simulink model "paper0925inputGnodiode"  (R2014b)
settings: Solver=ode15s  StartTime=0.0  StopTime=24  FixedStep=1e-4  RelTol=1e-3
libraries: nesl_utility x19, elec_lib x16, fl_lib x3

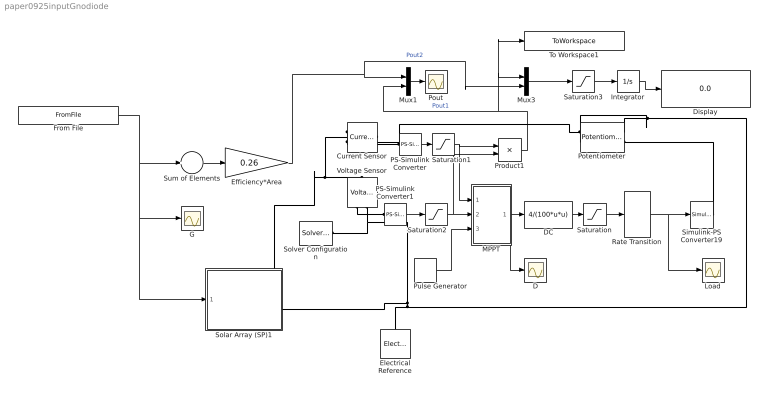
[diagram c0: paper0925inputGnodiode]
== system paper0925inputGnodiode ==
  Current Sensor : fl_lib/Electrical/Electrical Sensors/Current Sensor
  D : Scope
  DC : Fcn  Expr=4/(100*u*u)
  Display : Display
  Efficiency*Area : Gain  Gain=0.26
  Electrical Reference : fl_lib/Electrical/Electrical Elements/Electrical Reference
  From File : FromFile  FileName=Goverlap0_3.mat  SampleTime=0
  G : Scope
  Integrator : Integrator
  Load : Scope
  MPPT : Subsystem
  Mux1 : Mux  Inputs=2
  Mux3 : Mux  Inputs=2
  PS-Simulink Converter : nesl_utility/PS-Simulink Converter  PhysicalDomain=network_engine_domain  SubClassName=ps_output  LeftPortType=input  RightPortType=output  PseudoPeriodic=off  Frequencies=[]  Unit=1  AffineConversion=off
  PS-Simulink Converter1 : nesl_utility/PS-Simulink Converter  PhysicalDomain=network_engine_domain  SubClassName=ps_output  LeftPortType=input  RightPortType=output  PseudoPeriodic=off  Frequencies=[]  Unit=1  AffineConversion=off
  Potentiometer : elec_lib/Passive Devices/Potentiometer  R0=100 Ohm  Rw=0.01 Ohm  Rcenter=200 Ohm  xmin=0  xmax=1  Taper=1  Gradient=1  xminL=0  xmaxL=1  lambda=1  A=1 Ohm
  Pout : Scope
  Product1 : Product
  Pulse Generator : DiscretePulseGenerator  PulseType=Time based  Period=0.5  PulseWidth=0.1
  Rate Transition : RateTransition
  Saturation : Saturate  UpperLimit=1  LowerLimit=0
  Saturation1 : Saturate  UpperLimit=40  LowerLimit=0
  Saturation2 : Saturate  UpperLimit=500  LowerLimit=0
  Saturation3 : Saturate  UpperLimit=6000  LowerLimit=0
  Simulink-PS Converter19 : nesl_utility/Simulink-PS Converter  PhysicalDomain=network_engine_domain  SubClassName=ps_input  LeftPortType=input  RightPortType=output  PseudoPeriodic=off  Frequencies=[]  NoiseDistribution=none  NoiseParameters=[]  Unit=1  AffineConversion=off  InputFiltering=off  SimscapeFilterOrder=1  InputFilterTimeConstant=0.001  UdotUserProvided=1
  Solar Array (SP)1 : Subsystem
  Solver Configuration : nesl_utility/Solver Configuration  PhysicalDomain=network_engine_domain  SubClassName=solver  LeftPortType=input  RightPortType=generic  Accelerate=off  Tones=[]  Harmonics=[]  SimulateNoise=off  Profile=off  UseLocalSampling=off  EnableSwitchedLinearOptims=on  FrequencyDomain=off  UseCCode=off  RelTol=0.001  AbsTol=1e-06  MinStep=1e-09  ToWorkspace=off  DoDC=off  ResidualTolerance=1e-9  UseLocalSolver=on  LocalSolverChoice=NE_BACKWARD_EULER_ADVANCER  LocalSolverSampleTime=1e-4  DoFixedCost=on  MaxNonlinIter=3  MaxModeIter=2  LinearAlgebra=Sparse  DelaysMemoryBudget=1024  AutomaticFiltering=on  FilteringTimeConstant=0.001
  Sum of Elements : Sum  Inputs=+
  To Workspace1 : ToWorkspace  VariableName=Poverlap0_3SPnodiode  SampleTime=-1
  Voltage Sensor : fl_lib/Electrical/Electrical Sensors/Voltage Sensor
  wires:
  Sum of Elements/1 -> Efficiency*Area/1
  PS-Simulink Converter/1 -> Saturation1/1
  Product1/1 -> Mux3/1, To Workspace1/1, Mux1/2  "Pout1"
  PS-Simulink Converter1/1 -> Saturation2/1
  DC/1 -> Saturation/1
  Saturation/1 -> Rate Transition/1
  MPPT/1(D) -> D/1, DC/1
  Pulse Generator/1 -> MPPT/3(Control)
  Mux1/1 -> Pout/1
  Efficiency*Area/1 -> Mux3/2, Mux1/1  "Pout2"
  Mux3/1 -> Saturation3/1
  Rate Transition/1 -> Load/1, Simulink-PS Converter19/1
  From File/1 -> Solar Array (SP)1/1(G), G/1, Sum of Elements/1
  Saturation1/1 -> Product1/1, MPPT/1(I)
  Saturation2/1 -> Product1/2, MPPT/2(V)
  Saturation3/1 -> Integrator/1
  Integrator/1 -> Display/1
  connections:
  Voltage Sensor/LConn1 -- Solar Array (SP)1/RConn1 -- Current Sensor/LConn1
  Voltage Sensor/RConn2 -- Solar Array (SP)1/RConn2 -- Electrical Reference/LConn1 -- Potentiometer/LConn2 -- Potentiometer/RConn1 -- Solver Configuration/RConn1
  Current Sensor/RConn1 -- PS-Simulink Converter/LConn1
  Voltage Sensor/RConn1 -- PS-Simulink Converter1/LConn1
  Simulink-PS Converter19/RConn1 -- Potentiometer/RConn2
  Potentiometer/LConn1 -- Current Sensor/RConn2

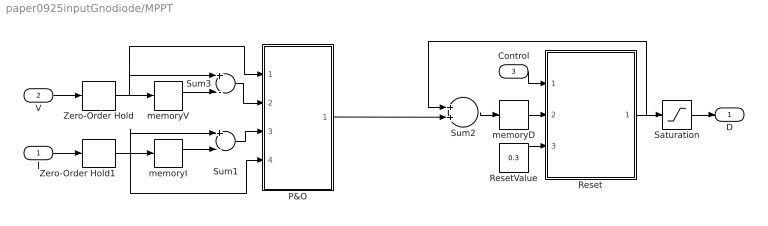
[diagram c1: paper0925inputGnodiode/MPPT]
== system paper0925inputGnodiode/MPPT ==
  I : Inport
  V : Inport  Port=2
  Control : Inport  Port=3
  P&O : MATLAB Function  TreatAsAtomicUnit=on
  Reset : MATLAB Function  TreatAsAtomicUnit=on
  ResetValue : Constant  Value=0.3
  Saturation : Saturate  UpperLimit=1  LowerLimit=1e-9
  Sum1 : Sum  Inputs=+-
  Sum2 : Sum  Inputs=2
  Sum3 : Sum  Inputs=+-
  Zero-Order Hold : ZeroOrderHold  SampleTime=1e-3
  Zero-Order Hold1 : ZeroOrderHold  SampleTime=1e-3
  memoryD : Memory  X0=0.3  InheritSampleTime=on
  memoryI : Memory  InheritSampleTime=on
  memoryV : Memory  InheritSampleTime=on
  D : Outport
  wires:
  Sum2/1 -> memoryD/1
  V/1 -> Zero-Order Hold/1
  I/1 -> Zero-Order Hold1/1
  Zero-Order Hold/1 -> P&O/1(V), Sum3/1, memoryV/1
  memoryV/1 -> Sum3/2
  Zero-Order Hold1/1 -> Sum1/1, P&O/4(I), memoryI/1
  memoryI/1 -> Sum1/2
  Saturation/1 -> D/1
  Sum3/1 -> P&O/2(dV)
  Sum1/1 -> P&O/3(dI)
  P&O/1(dD) -> Sum2/2
  ResetValue/1 -> Reset/3(ResetValue)
  memoryD/1 -> Reset/2(in)
  Reset/1(out) -> Sum2/1, Saturation/1
  Control/1 -> Reset/1(control)

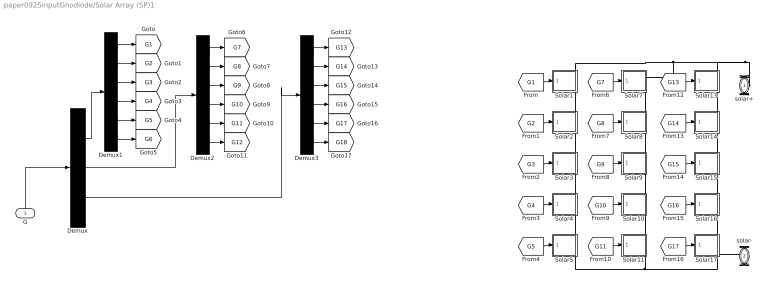
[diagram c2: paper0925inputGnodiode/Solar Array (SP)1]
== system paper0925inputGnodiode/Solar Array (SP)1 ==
  G : Inport
  Demux : Demux  Outputs=3
  Demux1 : Demux  Outputs=6
  Demux2 : Demux  Outputs=6
  Demux3 : Demux  Outputs=6
  Solar1 : Subsystem
  Solar10 : Subsystem
  Solar11 : Subsystem
  Solar13 : Subsystem
  Solar14 : Subsystem
  Solar15 : Subsystem
  Solar16 : Subsystem
  Solar17 : Subsystem
  Solar2 : Subsystem
  Solar3 : Subsystem
  Solar4 : Subsystem
  Solar5 : Subsystem
  Solar7 : Subsystem
  Solar8 : Subsystem
  Solar9 : Subsystem
  solar+ : PMIOPort  Port=1  Side=Right
  solar- : PMIOPort  Port=2  Side=Right
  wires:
  [G1] -> Solar1/1(G)
  [G2] -> Solar2/1(G)
  [G3] -> Solar3/1(G)
  G/1 -> Demux/1
  [G4] -> Solar4/1(G)
  [G5] -> Solar5/1(G)
  [G7] -> Solar7/1(G)
  [G8] -> Solar8/1(G)
  [G9] -> Solar9/1(G)
  [G10] -> Solar10/1(G)
  [G11] -> Solar11/1(G)
  [G13] -> Solar13/1(G)
  [G14] -> Solar14/1(G)
  [G15] -> Solar15/1(G)
  [G16] -> Solar16/1(G)
  [G17] -> Solar17/1(G)
  Demux/1 -> Demux1/1
  Demux1/1 -> [G1]
  Demux1/2 -> [G2]
  Demux1/3 -> [G3]
  Demux1/4 -> [G4]
  Demux1/5 -> [G5]
  Demux1/6 -> [G6]
  Demux/2 -> Demux2/1
  Demux/3 -> Demux3/1
  Demux2/1 -> [G7]
  Demux2/2 -> [G8]
  Demux2/3 -> [G9]
  Demux2/4 -> [G10]
  Demux2/5 -> [G11]
  Demux2/6 -> [G12]
  Demux3/1 -> [G13]
  Demux3/2 -> [G14]
  Demux3/3 -> [G15]
  Demux3/4 -> [G16]
  Demux3/5 -> [G17]
  Demux3/6 -> [G18]
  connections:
  Solar15/RConn2 -- Solar16/RConn1
  Solar13/RConn2 -- Solar14/RConn1
  Solar8/RConn2 -- Solar9/RConn1
  Solar4/RConn2 -- Solar5/RConn1
  Solar5/RConn2 -- Solar11/RConn2 -- Solar17/RConn2 -- solar-/RConn1
  solar+/RConn1 -- Solar1/RConn1 -- Solar7/RConn1 -- Solar13/RConn1
  Solar1/RConn2 -- Solar2/RConn1
  Solar7/RConn2 -- Solar8/RConn1
  Solar14/RConn2 -- Solar15/RConn1
  Solar2/RConn2 -- Solar3/RConn1
  Solar3/RConn2 -- Solar4/RConn1
  Solar9/RConn2 -- Solar10/RConn1
  Solar16/RConn2 -- Solar17/RConn1
  Solar10/RConn2 -- Solar11/RConn1

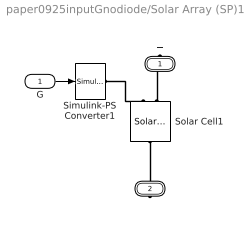
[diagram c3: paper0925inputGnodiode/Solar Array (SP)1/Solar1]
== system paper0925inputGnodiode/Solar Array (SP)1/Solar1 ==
  G : Inport
  Simulink-PS Converter1 : nesl_utility/Simulink-PS Converter  PhysicalDomain=network_engine_domain  SubClassName=ps_input  LeftPortType=input  RightPortType=output  PseudoPeriodic=off  Frequencies=[]  NoiseDistribution=none  NoiseParameters=[]  Unit=1  AffineConversion=off  InputFiltering=off  SimscapeFilterOrder=1  InputFilterTimeConstant=0.001  UdotUserProvided=1
  Solar Cell1 : elec_lib/Sources/Solar Cell  prm=1  Isc=7.34 A  Voc=0.6 V  Is=1e-6 A  Is2=0 A  Iph=7.34 A  Ir0=1000 W/m^2  ec=1.2  N2=2  Rs=1e-3 Ohm  Rp=Inf Ohm  N_series=90  TIPH1=0 1/K  EG=1.11 eV  TXIS1=3  TXIS2=3  TRS1=0  TRP1=0  Tmeas=25 C  TFIXED=25 C  thermal_mass=100 J/K  initial_temperature=25 C
  + : PMIOPort  Port=1  Side=Right
  - : PMIOPort  Port=2  Side=Right
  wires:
  G/1 -> Simulink-PS Converter1/1
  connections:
  Simulink-PS Converter1/RConn1 -- Solar Cell1/LConn1
  Solar Cell1/LConn2 -- +/RConn1
  Solar Cell1/RConn1 -- -/RConn1

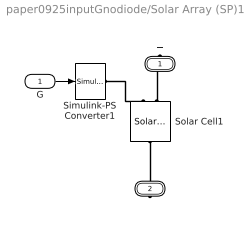
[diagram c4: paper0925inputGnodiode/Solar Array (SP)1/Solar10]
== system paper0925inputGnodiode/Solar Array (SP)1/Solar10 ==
  G : Inport
  Simulink-PS Converter1 : nesl_utility/Simulink-PS Converter  PhysicalDomain=network_engine_domain  SubClassName=ps_input  LeftPortType=input  RightPortType=output  PseudoPeriodic=off  Frequencies=[]  NoiseDistribution=none  NoiseParameters=[]  Unit=1  AffineConversion=off  InputFiltering=off  SimscapeFilterOrder=1  InputFilterTimeConstant=0.001  UdotUserProvided=1
  Solar Cell1 : elec_lib/Sources/Solar Cell  prm=1  Isc=7.34 A  Voc=0.6 V  Is=1e-6 A  Is2=0 A  Iph=7.34 A  Ir0=1000 W/m^2  ec=1.2  N2=2  Rs=1e-3 Ohm  Rp=Inf Ohm  N_series=90  TIPH1=0 1/K  EG=1.11 eV  TXIS1=3  TXIS2=3  TRS1=0  TRP1=0  Tmeas=25 C  TFIXED=25 C  thermal_mass=100 J/K  initial_temperature=25 C
  + : PMIOPort  Port=1  Side=Right
  - : PMIOPort  Port=2  Side=Right
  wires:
  G/1 -> Simulink-PS Converter1/1
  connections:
  Simulink-PS Converter1/RConn1 -- Solar Cell1/LConn1
  Solar Cell1/LConn2 -- +/RConn1
  Solar Cell1/RConn1 -- -/RConn1

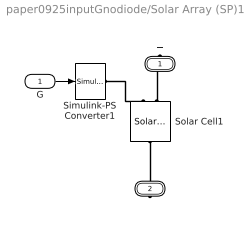
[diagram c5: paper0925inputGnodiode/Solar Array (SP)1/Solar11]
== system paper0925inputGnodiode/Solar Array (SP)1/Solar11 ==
  G : Inport
  Simulink-PS Converter1 : nesl_utility/Simulink-PS Converter  PhysicalDomain=network_engine_domain  SubClassName=ps_input  LeftPortType=input  RightPortType=output  PseudoPeriodic=off  Frequencies=[]  NoiseDistribution=none  NoiseParameters=[]  Unit=1  AffineConversion=off  InputFiltering=off  SimscapeFilterOrder=1  InputFilterTimeConstant=0.001  UdotUserProvided=1
  Solar Cell1 : elec_lib/Sources/Solar Cell  prm=1  Isc=7.34 A  Voc=0.6 V  Is=1e-6 A  Is2=0 A  Iph=7.34 A  Ir0=1000 W/m^2  ec=1.2  N2=2  Rs=1e-3 Ohm  Rp=Inf Ohm  N_series=90  TIPH1=0 1/K  EG=1.11 eV  TXIS1=3  TXIS2=3  TRS1=0  TRP1=0  Tmeas=25 C  TFIXED=25 C  thermal_mass=100 J/K  initial_temperature=25 C
  + : PMIOPort  Port=1  Side=Right
  - : PMIOPort  Port=2  Side=Right
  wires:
  G/1 -> Simulink-PS Converter1/1
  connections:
  Simulink-PS Converter1/RConn1 -- Solar Cell1/LConn1
  Solar Cell1/LConn2 -- +/RConn1
  Solar Cell1/RConn1 -- -/RConn1

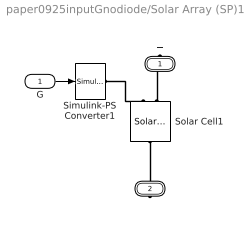
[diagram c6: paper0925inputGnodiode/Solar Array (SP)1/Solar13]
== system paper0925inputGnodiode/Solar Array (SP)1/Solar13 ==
  G : Inport
  Simulink-PS Converter1 : nesl_utility/Simulink-PS Converter  PhysicalDomain=network_engine_domain  SubClassName=ps_input  LeftPortType=input  RightPortType=output  PseudoPeriodic=off  Frequencies=[]  NoiseDistribution=none  NoiseParameters=[]  Unit=1  AffineConversion=off  InputFiltering=off  SimscapeFilterOrder=1  InputFilterTimeConstant=0.001  UdotUserProvided=1
  Solar Cell1 : elec_lib/Sources/Solar Cell  prm=1  Isc=7.34 A  Voc=0.6 V  Is=1e-6 A  Is2=0 A  Iph=7.34 A  Ir0=1000 W/m^2  ec=1.2  N2=2  Rs=1e-3 Ohm  Rp=Inf Ohm  N_series=90  TIPH1=0 1/K  EG=1.11 eV  TXIS1=3  TXIS2=3  TRS1=0  TRP1=0  Tmeas=25 C  TFIXED=25 C  thermal_mass=100 J/K  initial_temperature=25 C
  + : PMIOPort  Port=1  Side=Right
  - : PMIOPort  Port=2  Side=Right
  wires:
  G/1 -> Simulink-PS Converter1/1
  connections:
  Simulink-PS Converter1/RConn1 -- Solar Cell1/LConn1
  Solar Cell1/LConn2 -- +/RConn1
  Solar Cell1/RConn1 -- -/RConn1

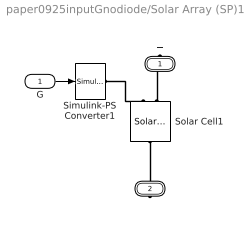
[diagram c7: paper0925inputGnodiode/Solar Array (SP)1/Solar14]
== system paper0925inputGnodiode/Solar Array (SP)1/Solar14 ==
  G : Inport
  Simulink-PS Converter1 : nesl_utility/Simulink-PS Converter  PhysicalDomain=network_engine_domain  SubClassName=ps_input  LeftPortType=input  RightPortType=output  PseudoPeriodic=off  Frequencies=[]  NoiseDistribution=none  NoiseParameters=[]  Unit=1  AffineConversion=off  InputFiltering=off  SimscapeFilterOrder=1  InputFilterTimeConstant=0.001  UdotUserProvided=1
  Solar Cell1 : elec_lib/Sources/Solar Cell  prm=1  Isc=7.34 A  Voc=0.6 V  Is=1e-6 A  Is2=0 A  Iph=7.34 A  Ir0=1000 W/m^2  ec=1.2  N2=2  Rs=1e-3 Ohm  Rp=Inf Ohm  N_series=90  TIPH1=0 1/K  EG=1.11 eV  TXIS1=3  TXIS2=3  TRS1=0  TRP1=0  Tmeas=25 C  TFIXED=25 C  thermal_mass=100 J/K  initial_temperature=25 C
  + : PMIOPort  Port=1  Side=Right
  - : PMIOPort  Port=2  Side=Right
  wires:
  G/1 -> Simulink-PS Converter1/1
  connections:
  Simulink-PS Converter1/RConn1 -- Solar Cell1/LConn1
  Solar Cell1/LConn2 -- +/RConn1
  Solar Cell1/RConn1 -- -/RConn1

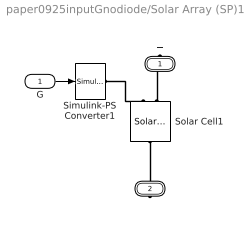
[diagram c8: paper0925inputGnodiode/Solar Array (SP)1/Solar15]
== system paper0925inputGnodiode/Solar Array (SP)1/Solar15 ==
  G : Inport
  Simulink-PS Converter1 : nesl_utility/Simulink-PS Converter  PhysicalDomain=network_engine_domain  SubClassName=ps_input  LeftPortType=input  RightPortType=output  PseudoPeriodic=off  Frequencies=[]  NoiseDistribution=none  NoiseParameters=[]  Unit=1  AffineConversion=off  InputFiltering=off  SimscapeFilterOrder=1  InputFilterTimeConstant=0.001  UdotUserProvided=1
  Solar Cell1 : elec_lib/Sources/Solar Cell  prm=1  Isc=7.34 A  Voc=0.6 V  Is=1e-6 A  Is2=0 A  Iph=7.34 A  Ir0=1000 W/m^2  ec=1.2  N2=2  Rs=1e-3 Ohm  Rp=Inf Ohm  N_series=90  TIPH1=0 1/K  EG=1.11 eV  TXIS1=3  TXIS2=3  TRS1=0  TRP1=0  Tmeas=25 C  TFIXED=25 C  thermal_mass=100 J/K  initial_temperature=25 C
  + : PMIOPort  Port=1  Side=Right
  - : PMIOPort  Port=2  Side=Right
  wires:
  G/1 -> Simulink-PS Converter1/1
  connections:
  Simulink-PS Converter1/RConn1 -- Solar Cell1/LConn1
  Solar Cell1/LConn2 -- +/RConn1
  Solar Cell1/RConn1 -- -/RConn1

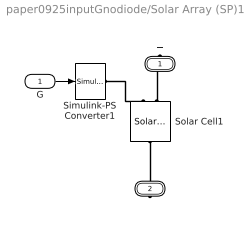
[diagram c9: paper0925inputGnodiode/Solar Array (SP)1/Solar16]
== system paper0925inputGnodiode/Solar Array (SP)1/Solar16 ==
  G : Inport
  Simulink-PS Converter1 : nesl_utility/Simulink-PS Converter  PhysicalDomain=network_engine_domain  SubClassName=ps_input  LeftPortType=input  RightPortType=output  PseudoPeriodic=off  Frequencies=[]  NoiseDistribution=none  NoiseParameters=[]  Unit=1  AffineConversion=off  InputFiltering=off  SimscapeFilterOrder=1  InputFilterTimeConstant=0.001  UdotUserProvided=1
  Solar Cell1 : elec_lib/Sources/Solar Cell  prm=1  Isc=7.34 A  Voc=0.6 V  Is=1e-6 A  Is2=0 A  Iph=7.34 A  Ir0=1000 W/m^2  ec=1.2  N2=2  Rs=1e-3 Ohm  Rp=Inf Ohm  N_series=90  TIPH1=0 1/K  EG=1.11 eV  TXIS1=3  TXIS2=3  TRS1=0  TRP1=0  Tmeas=25 C  TFIXED=25 C  thermal_mass=100 J/K  initial_temperature=25 C
  + : PMIOPort  Port=1  Side=Right
  - : PMIOPort  Port=2  Side=Right
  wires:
  G/1 -> Simulink-PS Converter1/1
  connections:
  Simulink-PS Converter1/RConn1 -- Solar Cell1/LConn1
  Solar Cell1/LConn2 -- +/RConn1
  Solar Cell1/RConn1 -- -/RConn1

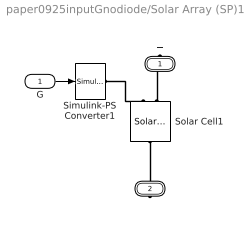
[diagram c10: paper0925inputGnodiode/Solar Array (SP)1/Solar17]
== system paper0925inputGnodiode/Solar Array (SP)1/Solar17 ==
  G : Inport
  Simulink-PS Converter1 : nesl_utility/Simulink-PS Converter  PhysicalDomain=network_engine_domain  SubClassName=ps_input  LeftPortType=input  RightPortType=output  PseudoPeriodic=off  Frequencies=[]  NoiseDistribution=none  NoiseParameters=[]  Unit=1  AffineConversion=off  InputFiltering=off  SimscapeFilterOrder=1  InputFilterTimeConstant=0.001  UdotUserProvided=1
  Solar Cell1 : elec_lib/Sources/Solar Cell  prm=1  Isc=7.34 A  Voc=0.6 V  Is=1e-6 A  Is2=0 A  Iph=7.34 A  Ir0=1000 W/m^2  ec=1.2  N2=2  Rs=1e-3 Ohm  Rp=Inf Ohm  N_series=90  TIPH1=0 1/K  EG=1.11 eV  TXIS1=3  TXIS2=3  TRS1=0  TRP1=0  Tmeas=25 C  TFIXED=25 C  thermal_mass=100 J/K  initial_temperature=25 C
  + : PMIOPort  Port=1  Side=Right
  - : PMIOPort  Port=2  Side=Right
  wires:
  G/1 -> Simulink-PS Converter1/1
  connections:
  Simulink-PS Converter1/RConn1 -- Solar Cell1/LConn1
  Solar Cell1/LConn2 -- +/RConn1
  Solar Cell1/RConn1 -- -/RConn1

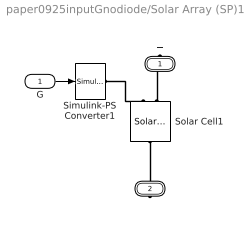
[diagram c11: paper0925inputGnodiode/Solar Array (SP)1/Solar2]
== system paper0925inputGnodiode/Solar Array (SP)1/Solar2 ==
  G : Inport
  Simulink-PS Converter1 : nesl_utility/Simulink-PS Converter  PhysicalDomain=network_engine_domain  SubClassName=ps_input  LeftPortType=input  RightPortType=output  PseudoPeriodic=off  Frequencies=[]  NoiseDistribution=none  NoiseParameters=[]  Unit=1  AffineConversion=off  InputFiltering=off  SimscapeFilterOrder=1  InputFilterTimeConstant=0.001  UdotUserProvided=1
  Solar Cell1 : elec_lib/Sources/Solar Cell  prm=1  Isc=7.34 A  Voc=0.6 V  Is=1e-6 A  Is2=0 A  Iph=7.34 A  Ir0=1000 W/m^2  ec=1.2  N2=2  Rs=1e-3 Ohm  Rp=Inf Ohm  N_series=90  TIPH1=0 1/K  EG=1.11 eV  TXIS1=3  TXIS2=3  TRS1=0  TRP1=0  Tmeas=25 C  TFIXED=25 C  thermal_mass=100 J/K  initial_temperature=25 C
  + : PMIOPort  Port=1  Side=Right
  - : PMIOPort  Port=2  Side=Right
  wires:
  G/1 -> Simulink-PS Converter1/1
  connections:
  Simulink-PS Converter1/RConn1 -- Solar Cell1/LConn1
  Solar Cell1/LConn2 -- +/RConn1
  Solar Cell1/RConn1 -- -/RConn1

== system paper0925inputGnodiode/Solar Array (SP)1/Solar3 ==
  G : Inport
  Simulink-PS Converter1 : nesl_utility/Simulink-PS Converter  PhysicalDomain=network_engine_domain  SubClassName=ps_input  LeftPortType=input  RightPortType=output  PseudoPeriodic=off  Frequencies=[]  NoiseDistribution=none  NoiseParameters=[]  Unit=1  AffineConversion=off  InputFiltering=off  SimscapeFilterOrder=1  InputFilterTimeConstant=0.001  UdotUserProvided=1
  Solar Cell1 : elec_lib/Sources/Solar Cell  prm=1  Isc=7.34 A  Voc=0.6 V  Is=1e-6 A  Is2=0 A  Iph=7.34 A  Ir0=1000 W/m^2  ec=1.2  N2=2  Rs=1e-3 Ohm  Rp=Inf Ohm  N_series=90  TIPH1=0 1/K  EG=1.11 eV  TXIS1=3  TXIS2=3  TRS1=0  TRP1=0  Tmeas=25 C  TFIXED=25 C  thermal_mass=100 J/K  initial_temperature=25 C
  + : PMIOPort  Port=1  Side=Right
  - : PMIOPort  Port=2  Side=Right
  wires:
  G/1 -> Simulink-PS Converter1/1
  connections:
  Simulink-PS Converter1/RConn1 -- Solar Cell1/LConn1
  Solar Cell1/LConn2 -- +/RConn1
  Solar Cell1/RConn1 -- -/RConn1

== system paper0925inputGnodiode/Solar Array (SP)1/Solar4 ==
  G : Inport
  Simulink-PS Converter1 : nesl_utility/Simulink-PS Converter  PhysicalDomain=network_engine_domain  SubClassName=ps_input  LeftPortType=input  RightPortType=output  PseudoPeriodic=off  Frequencies=[]  NoiseDistribution=none  NoiseParameters=[]  Unit=1  AffineConversion=off  InputFiltering=off  SimscapeFilterOrder=1  InputFilterTimeConstant=0.001  UdotUserProvided=1
  Solar Cell1 : elec_lib/Sources/Solar Cell  prm=1  Isc=7.34 A  Voc=0.6 V  Is=1e-6 A  Is2=0 A  Iph=7.34 A  Ir0=1000 W/m^2  ec=1.2  N2=2  Rs=1e-3 Ohm  Rp=Inf Ohm  N_series=90  TIPH1=0 1/K  EG=1.11 eV  TXIS1=3  TXIS2=3  TRS1=0  TRP1=0  Tmeas=25 C  TFIXED=25 C  thermal_mass=100 J/K  initial_temperature=25 C
  + : PMIOPort  Port=1  Side=Right
  - : PMIOPort  Port=2  Side=Right
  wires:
  G/1 -> Simulink-PS Converter1/1
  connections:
  Simulink-PS Converter1/RConn1 -- Solar Cell1/LConn1
  Solar Cell1/LConn2 -- +/RConn1
  Solar Cell1/RConn1 -- -/RConn1

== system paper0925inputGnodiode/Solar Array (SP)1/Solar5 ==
  G : Inport
  Simulink-PS Converter1 : nesl_utility/Simulink-PS Converter  PhysicalDomain=network_engine_domain  SubClassName=ps_input  LeftPortType=input  RightPortType=output  PseudoPeriodic=off  Frequencies=[]  NoiseDistribution=none  NoiseParameters=[]  Unit=1  AffineConversion=off  InputFiltering=off  SimscapeFilterOrder=1  InputFilterTimeConstant=0.001  UdotUserProvided=1
  Solar Cell1 : elec_lib/Sources/Solar Cell  prm=1  Isc=7.34 A  Voc=0.6 V  Is=1e-6 A  Is2=0 A  Iph=7.34 A  Ir0=1000 W/m^2  ec=1.2  N2=2  Rs=1e-3 Ohm  Rp=Inf Ohm  N_series=90  TIPH1=0 1/K  EG=1.11 eV  TXIS1=3  TXIS2=3  TRS1=0  TRP1=0  Tmeas=25 C  TFIXED=25 C  thermal_mass=100 J/K  initial_temperature=25 C
  + : PMIOPort  Port=1  Side=Right
  - : PMIOPort  Port=2  Side=Right
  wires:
  G/1 -> Simulink-PS Converter1/1
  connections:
  Simulink-PS Converter1/RConn1 -- Solar Cell1/LConn1
  Solar Cell1/LConn2 -- +/RConn1
  Solar Cell1/RConn1 -- -/RConn1

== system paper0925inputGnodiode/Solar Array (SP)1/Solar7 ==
  G : Inport
  Simulink-PS Converter1 : nesl_utility/Simulink-PS Converter  PhysicalDomain=network_engine_domain  SubClassName=ps_input  LeftPortType=input  RightPortType=output  PseudoPeriodic=off  Frequencies=[]  NoiseDistribution=none  NoiseParameters=[]  Unit=1  AffineConversion=off  InputFiltering=off  SimscapeFilterOrder=1  InputFilterTimeConstant=0.001  UdotUserProvided=1
  Solar Cell1 : elec_lib/Sources/Solar Cell  prm=1  Isc=7.34 A  Voc=0.6 V  Is=1e-6 A  Is2=0 A  Iph=7.34 A  Ir0=1000 W/m^2  ec=1.2  N2=2  Rs=1e-3 Ohm  Rp=Inf Ohm  N_series=90  TIPH1=0 1/K  EG=1.11 eV  TXIS1=3  TXIS2=3  TRS1=0  TRP1=0  Tmeas=25 C  TFIXED=25 C  thermal_mass=100 J/K  initial_temperature=25 C
  + : PMIOPort  Port=1  Side=Right
  - : PMIOPort  Port=2  Side=Right
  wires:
  G/1 -> Simulink-PS Converter1/1
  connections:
  Simulink-PS Converter1/RConn1 -- Solar Cell1/LConn1
  Solar Cell1/LConn2 -- +/RConn1
  Solar Cell1/RConn1 -- -/RConn1

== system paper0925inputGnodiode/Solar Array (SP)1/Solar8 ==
  G : Inport
  Simulink-PS Converter1 : nesl_utility/Simulink-PS Converter  PhysicalDomain=network_engine_domain  SubClassName=ps_input  LeftPortType=input  RightPortType=output  PseudoPeriodic=off  Frequencies=[]  NoiseDistribution=none  NoiseParameters=[]  Unit=1  AffineConversion=off  InputFiltering=off  SimscapeFilterOrder=1  InputFilterTimeConstant=0.001  UdotUserProvided=1
  Solar Cell1 : elec_lib/Sources/Solar Cell  prm=1  Isc=7.34 A  Voc=0.6 V  Is=1e-6 A  Is2=0 A  Iph=7.34 A  Ir0=1000 W/m^2  ec=1.2  N2=2  Rs=1e-3 Ohm  Rp=Inf Ohm  N_series=90  TIPH1=0 1/K  EG=1.11 eV  TXIS1=3  TXIS2=3  TRS1=0  TRP1=0  Tmeas=25 C  TFIXED=25 C  thermal_mass=100 J/K  initial_temperature=25 C
  + : PMIOPort  Port=1  Side=Right
  - : PMIOPort  Port=2  Side=Right
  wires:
  G/1 -> Simulink-PS Converter1/1
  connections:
  Simulink-PS Converter1/RConn1 -- Solar Cell1/LConn1
  Solar Cell1/LConn2 -- +/RConn1
  Solar Cell1/RConn1 -- -/RConn1

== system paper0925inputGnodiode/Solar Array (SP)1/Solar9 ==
  G : Inport
  Simulink-PS Converter1 : nesl_utility/Simulink-PS Converter  PhysicalDomain=network_engine_domain  SubClassName=ps_input  LeftPortType=input  RightPortType=output  PseudoPeriodic=off  Frequencies=[]  NoiseDistribution=none  NoiseParameters=[]  Unit=1  AffineConversion=off  InputFiltering=off  SimscapeFilterOrder=1  InputFilterTimeConstant=0.001  UdotUserProvided=1
  Solar Cell1 : elec_lib/Sources/Solar Cell  prm=1  Isc=7.34 A  Voc=0.6 V  Is=1e-6 A  Is2=0 A  Iph=7.34 A  Ir0=1000 W/m^2  ec=1.2  N2=2  Rs=1e-3 Ohm  Rp=Inf Ohm  N_series=90  TIPH1=0 1/K  EG=1.11 eV  TXIS1=3  TXIS2=3  TRS1=0  TRP1=0  Tmeas=25 C  TFIXED=25 C  thermal_mass=100 J/K  initial_temperature=25 C
  + : PMIOPort  Port=1  Side=Right
  - : PMIOPort  Port=2  Side=Right
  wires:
  G/1 -> Simulink-PS Converter1/1
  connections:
  Simulink-PS Converter1/RConn1 -- Solar Cell1/LConn1
  Solar Cell1/LConn2 -- +/RConn1
  Solar Cell1/RConn1 -- -/RConn1

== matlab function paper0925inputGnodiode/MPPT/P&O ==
function dD  = fcn(V,dV,dI,I)
%#codegen
step=0.001;

dP=(V+dV).*(I+dI)-V.*I;
if abs(dP) > 1e-6
    if dP < 0
        if dV < 0
            dD = -step;
        else
            dD = step;
        end
    else
        if dV < 0
            dD = step;
        else
            dD = -step;
        end
    end
else dD=0;
end

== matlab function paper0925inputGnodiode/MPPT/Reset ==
function out  = fcn(control,in,ResetValue)
%#codegen

if control ==1
    out=ResetValue;
else
    out=in;
end
